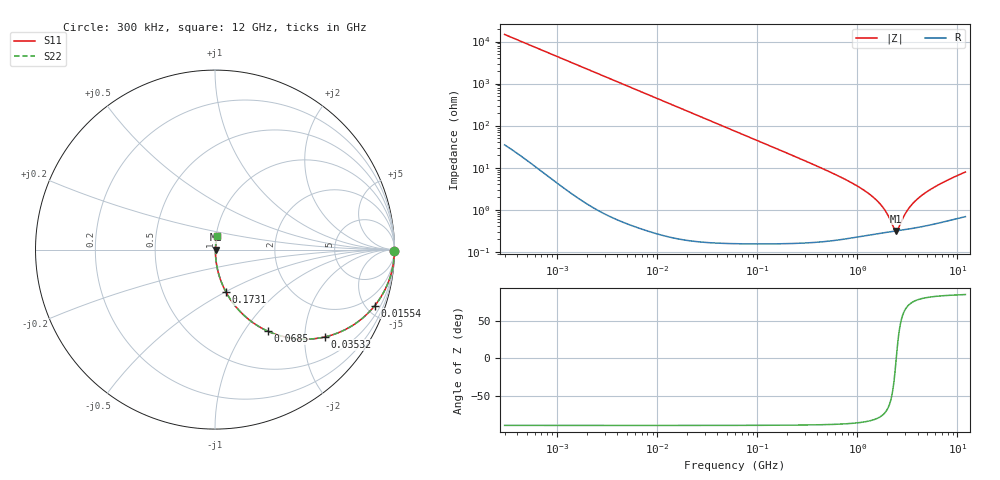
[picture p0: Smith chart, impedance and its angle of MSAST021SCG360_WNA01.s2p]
! MSAST021SCG360_WNA01  S-PARAMETER MODEL  ( Standard Model )
! Model Generated by TAIYO YUDEN Corporation (http://www.ty-top.com)
! Version 2.0
! TAIYO YUDEN Control No. 231201
! Copyright(c) 2023 TAIYO YUDEN CO.,LTD. All Rights Reserved.
! Product Description (link to TY-COMPAS)
! https://ds.yuden.co.jp/TYCOMPAS/or/detail?pn=MSAST021SCG360JWNA01&u=M
! Products Name : Multilayer Ceramic Capacitors
! Characteristics :
!  Capacitance : 36 [pF] , Rated Voltage : 25 [V] , TCC : CG / C0G
!  Case Size : 0.25 x 0.125 / 0.0098 x 0.0049 [mm/inch] , Thickness : 0.125 / 0.0049 [mm/inch]
!  (Conditions: Temperature = 25 [degC] , DC Bias Voltage = 0 [V])
! External Node Assignments :
!  1  o---| |---o  2
! GND o---------o GND
! Frequency Range : 0.3MHz  -  12000MHz  [ 401 STEP ]
# MHZ S RI R 50
! Freq[MHz].  S11 Real  S11 Imag  S21 Real  S21 Imag  S12 Real  S12 Imag  S22 Real  S22 Imag
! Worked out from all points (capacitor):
!   401 points, 300 kHz to 12 GHz, reference 50 ohm
!   read as one part in series: C = 36 pF near 316.3 kHz
!   lowest |Z| = 311 mohm at 2.448 GHz (marker M1)
!   series resonance near 2.448 GHz, so ESL is about 120 pH
!   S11 on the Smith chart (normalised r, x): 300 kHz: open; 15.54 MHz: 1.00, -5.70; 35.32 MHz: 1.00, -2.51; 68.5 MHz: 1.00, -1.29; 173.1 MHz: 1.00, -0.51; 12 GHz: 1.01, +0.16
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0.3  0.9999 -0.00679  6.2e-05 0.00679  6.2e-05 0.00679  0.9999 -0.00679
1.769972  0.9984 -0.0399  0.00162 0.0399  0.00162 0.0399  0.9984 -0.0399
4.716902  0.9887 -0.1053  0.0113 0.1053  0.0113 0.1053  0.9887 -0.1053
10.44266  0.9472 -0.2234  0.0528 0.2234  0.0528 0.2234  0.9472 -0.2234
15.53777  0.8902 -0.3123  0.1098 0.3123  0.1098 0.3123  0.8902 -0.3123
35.32224  0.6109 -0.4869  0.3891 0.4869  0.3891 0.4869  0.6109 -0.4869
60  0.3526 -0.4767  0.6474 0.4767  0.6474 0.4767  0.3526 -0.4767
68.49786  0.2948 -0.4548  0.7052 0.4548  0.7052 0.4548  0.2948 -0.4548
107.4644  0.1455 -0.3508  0.8545 0.3508  0.8545 0.3508  0.1455 -0.3508
173.124  0.062 -0.2382  0.938 0.2382  0.938 0.2382  0.062 -0.2382
353.9943  0.0163 -0.1199  0.9837 0.1199  0.9837 0.1199  0.0163 -0.1199
763.2128  0.00467 -0.0515  0.9953 0.0515  0.9953 0.0515  0.00467 -0.0515
1229.528  0.00311 -0.0263  0.9969 0.0263  0.9969 0.0263  0.00311 -0.0263
1689.663  0.0029 -0.0133  0.9971 0.0133  0.9971 0.0133  0.0029 -0.0133
2088.533  0.00297 -0.00557  0.997 0.00557  0.997 0.00557  0.00297 -0.00557
2321.999  0.00305 -0.00185  0.9969 0.00185  0.9969 0.00185  0.00305 -0.00185
2448.343  0.0031 5.39e-07  0.9969 -5.39e-07  0.9969 -5.39e-07  0.0031 5.39e-07
2581.562  0.00317 0.00184  0.9968 -0.00184  0.9968 -0.00184  0.00317 0.00184
3276.641  0.00356 0.0102  0.9964 -0.0102  0.9964 -0.0102  0.00356 0.0102
4158.869  0.00418 0.0191  0.9958 -0.0191  0.9958 -0.0191  0.00418 0.0191
6354.153  0.00612 0.0374  0.9939 -0.0374  0.9939 -0.0374  0.00612 0.0374
12000  0.0128 0.0769  0.9872 -0.0769  0.9872 -0.0769  0.0128 0.0769
